PROGRAM p06_ST_rtrig
VAR
	preklopnik: BOOL;
	lucka: BOOL;
	tipka1: BOOL;
	tipka2: BOOL;
	tipka: BOOL;
	tipkaStaro: BOOL;
END_VAR

// Detekcija pozitivne fronte na tipki
IF tipka AND NOT tipkaStaro THEN
	// Ob pozitivni fronti obrnemo stanje lucke
	lucka := NOT lucka;
	// Izpustimo ELSE, da povzročimo pomnjenje
END_IF

// Posodobimo staro stanje tipke
tipkaStaro := tipka;

END_PROGRAM
